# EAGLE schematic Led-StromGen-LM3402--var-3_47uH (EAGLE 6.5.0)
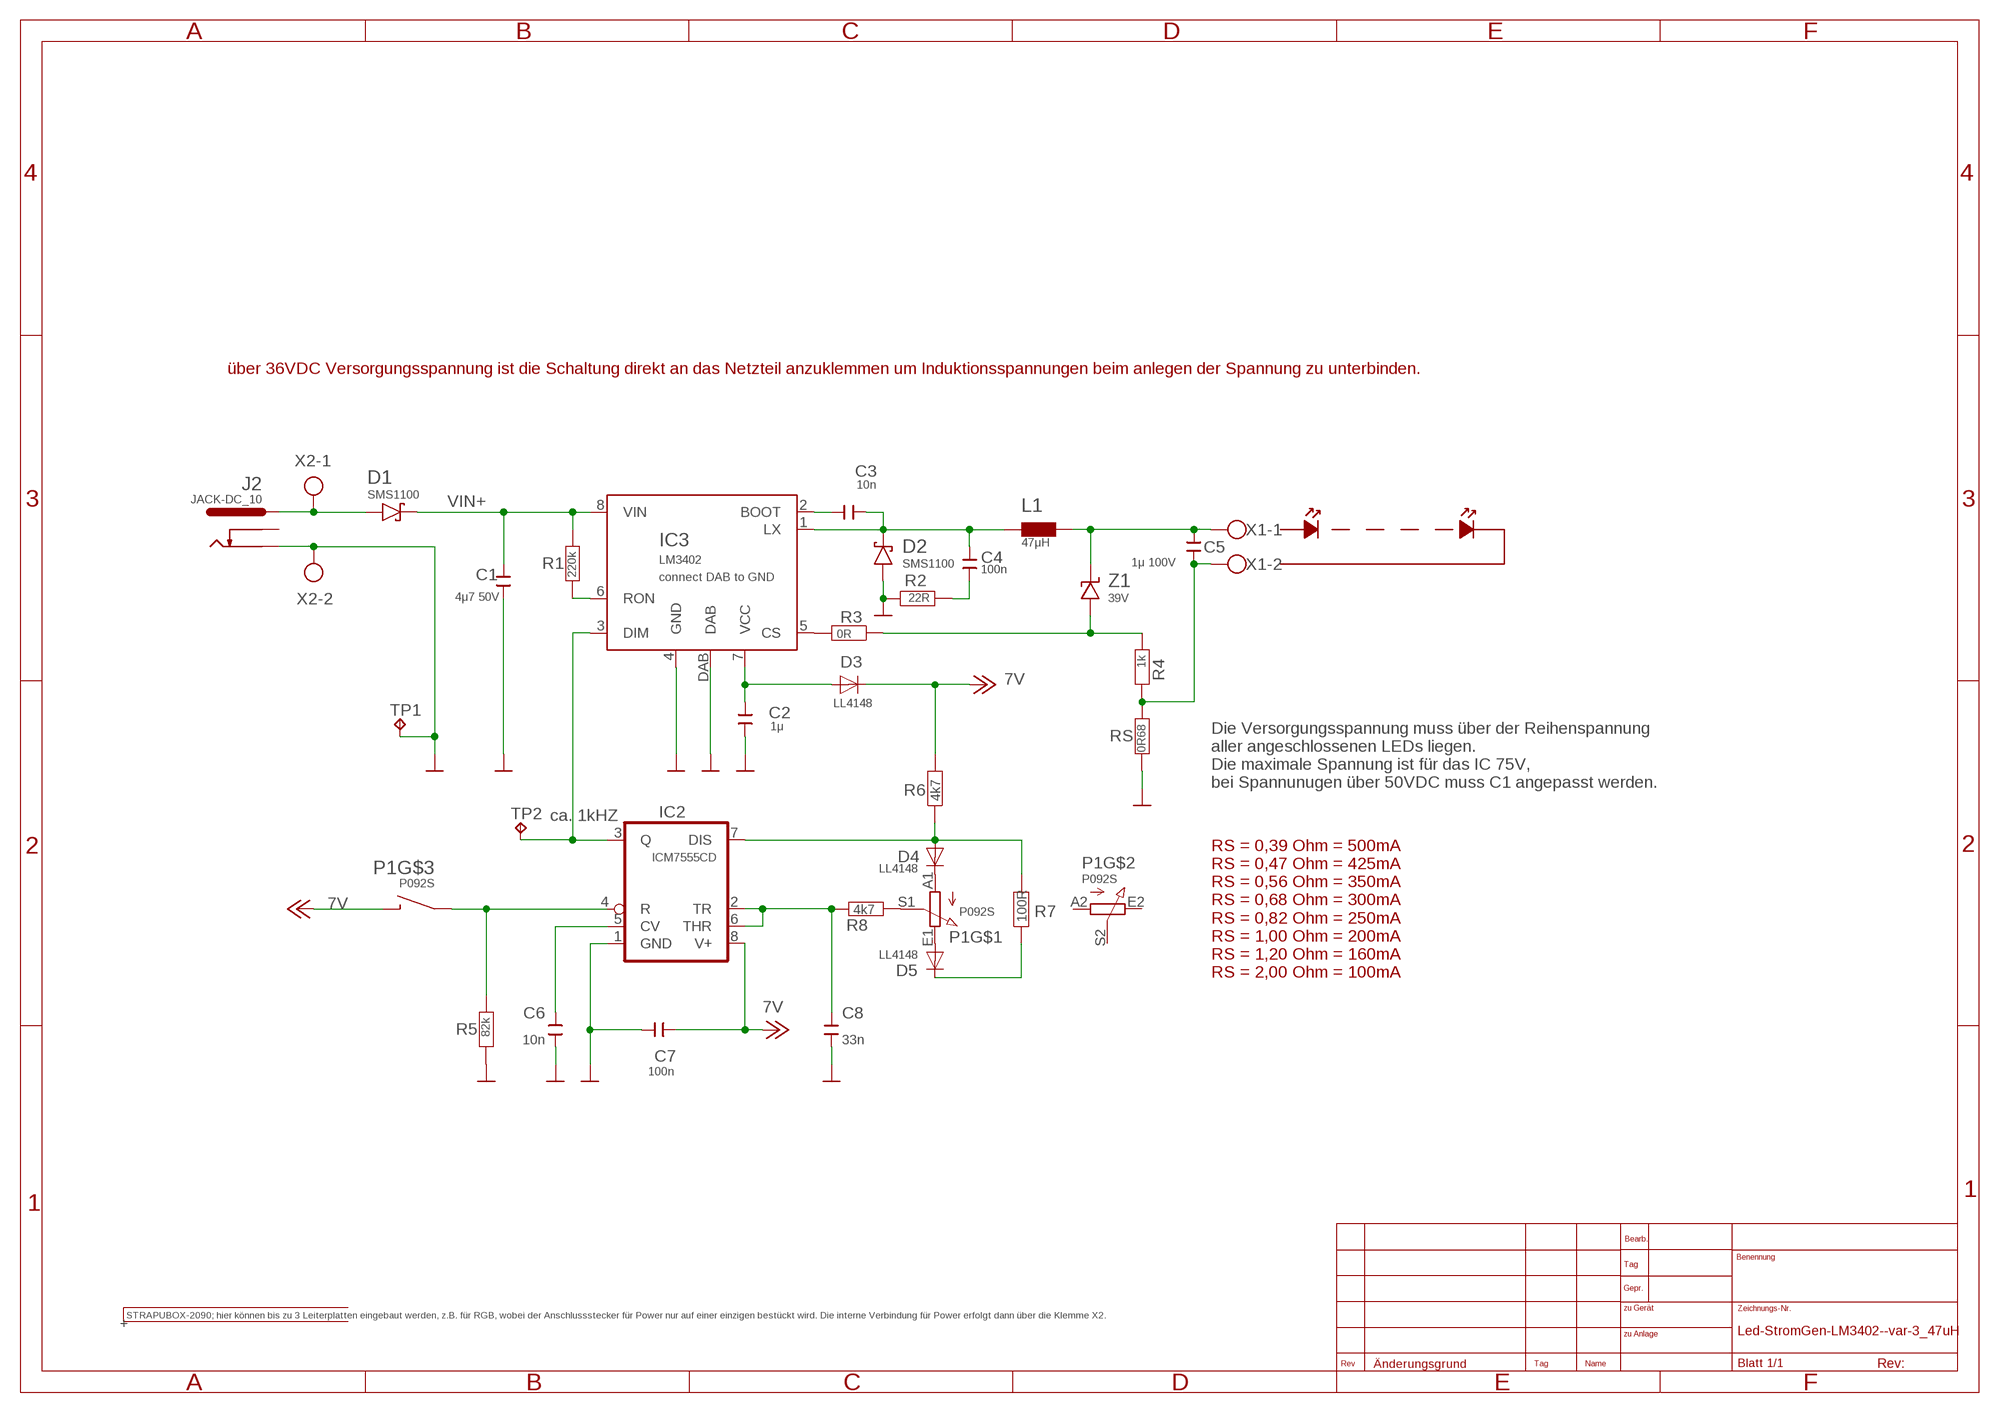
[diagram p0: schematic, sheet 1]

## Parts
BOX1  STRAPUBOX-2090; hier können bis zu 3 Leiterplatten eingebaut werden, z.B. für RGB, wobei der Anschlussstecker für Power nur auf einer einzigen bestückt wird. Die interne Verbindung für Power erfolgt dann über die Klemme X2.  STRAPUBOX-2090  [STRAPUBOX-2090]
C1  4μ7 50V  C-EUC1210K  [C1210K]
C2  1μ  C-EUC1206  [C1206]
C3  10n  C-EUC1206  [C1206]
C4  100n  C-EUC1206  [C1206]
C5  1μ 100V  C-EUC1210  [C1210]
C6  10n  C-EUC1206  [C1206]
C7  100n  C-EUC1206  [C1206]
C8  33n  C-EUC1206  [C1206]
D1  SMS1100  [MINI_MELF-0207R]
D2  SMS1100  [MINI_MELF-0207R]
D3  LL4148  LL4148MINIMELF  [MINIMELF]
D4  LL4148  LL4148MINIMELF  [MINIMELF]
D5  LL4148  LL4148MINIMELF  [MINIMELF]
IC2  ICM7555CD  NE555D  [SO08]
IC3  LM3402  [MSOP8]
J2  JACK-DC_10  [JACK-DC_10]
L1  47μH  B82464...  [B82464...]
P1  P092S  [P092S]
R1  220k  R-EU_R1206  [1206]
R2  22R  R-EU_R1206  [1206]
R3  0R  R-EU_R1206  [1206]
R4  1k  R-EU_R1206  [1206]
R5  82k  R-EU_R1206  [1206]
R6  4k7  R-EU_R1206  [1206]
R7  100R  R-EU_R1206  [1206]
R8  4k7  R-EU_R1206  [1206]
RS  0R68  R-EU_MELF0207R  [MINI_MELF-0207R]
TP1  GND  TP20SQ  [TP20SQ]
TP2  PWM  TP20SQ  [TP20SQ]
X1  AK500/2  [AK500/2]
X2  AK500/2  [AK500/2]
Z1  39V  ZMM  [MELF-LM34]

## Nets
7V: C7.1 D3.C IC2.8(V+) P1.SW1 R6.2 ; supply symbol labelled +12V, 7v
GND: C1.2 C2.2 C6.2 C7.2 C8.2 D2.2(A) IC2.1(GND) IC3.4(GND) IC3.DAB J2.SLIDE(SIDE) R2.1 R5.1 RS.1 TP1.TP X2.2
N$1: IC3.5(CS) R3.2
N$2: C4.2 R2.2
N$3: C3.2 C4.1 D2.1(C) IC3.1(LX) L1.1
N$4: IC3.6(RON) R1.1
N$5: C5.1 L1.2 X1.1 Z1.1(C)
N$6: C5.2 R4.1 RS.2 X1.2
N$7: D1.2(A) J2.PIN X2.1
N$8: C3.1 IC3.2(BOOT)
N$9: C2.1 D3.A IC3.7(VCC)
N$10: R3.1 R4.2 Z1.2(A)
N$11: P1.S1(S) R8.2
N$13: C8.1 IC2.2(TR) IC2.6(THR) R8.1
N$14: C6.1 IC2.5(CV)
N$20: D4.A IC2.7(DIS) R6.1 R7.2
N$22: D5.A P1.E1(E)
N$33: D4.C P1.A1(A)
N$53: D5.C R7.1
ON-OFF: IC2.4(R) P1.SW R5.2
PWM: IC2.3(Q) IC3.3(DIM) TP2.TP
VIN+: C1.1 D1.1(C) IC3.8(VIN) R1.2
Unconnected: J2.SW P1.A2(A) P1.E2(E) P1.S2(S)

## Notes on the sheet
- über 36VDC Versorgungsspannung ist die Schaltung direkt an das Netzteil anzuklemmen um Induktionsspannungen beim anlegen der Spannung zu unterbinden.
- Die Versorgungsspannung muss über der Reihenspannung 
  aller angeschlossenen LEDs liegen. 
  Die maximale Spannung ist für das IC 75V, 
  bei Spannunugen über 50VDC muss C1 angepasst werden.
- ca. 1kHZ
- RS = 0,39 Ohm = 500mA
  RS = 0,47 Ohm = 425mA
  RS = 0,56 Ohm = 350mA
  RS = 0,68 Ohm = 300mA
  RS = 0,82 Ohm = 250mA
  RS = 1,00 Ohm = 200mA
  RS = 1,20 Ohm = 160mA
  RS = 2,00 Ohm = 100mA

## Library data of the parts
BOX1 = Enclosures-DIN-Rail+more_1:STRAPUBOX-2090: STRABUBOX
C1 = rcl:C-EU: CAPACITOR, European symbol; OPTION: bis 50V
C2-C8 = rcl:C-EU: CAPACITOR, European symbol
D1 D2 = LED-Treiber:SMS1100
D3-D5 = SMD-rcldf_led:LL4148
IC2 = linear:*555: TIMER
IC3 = LED-Treiber:LM3402: 0.5A Constant Current Buck Regulator for Driving High Power LEDs 6-75V Connect DAB to GND
J2 = allgem:JACK-DC_10
L1 = inductor-fastron:B82464...; BUERKLIN-73D90--: 1uH bis 1000uH
P1 = pot:P092S
R1-R8 RS = rcl:R-EU_: RESISTOR, European symbol
TP1 TP2 = testpad:TP20SQ: TEST PIN
X1 X2 = con-ptr500:AK500/2: CONNECTOR
Z1 = allgem:ZMM; BUERKLIN-25S7360: 500mW mini-MELF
